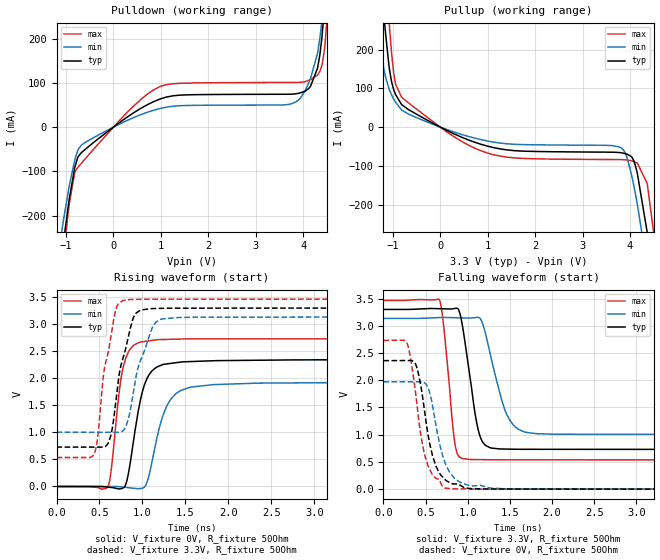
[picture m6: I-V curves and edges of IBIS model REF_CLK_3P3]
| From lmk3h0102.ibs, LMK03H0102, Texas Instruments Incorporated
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[Model]   REF_CLK_3P3
Model_type   Output
Polarity   Non-Inverting
Vmeas = 1.65
Vref = 0
Cref = 5pF
Rref = 100000
|   typ   min   max
C_comp   2.5pF   2pF   3pF
[Voltage Range]   3.3   3.135   3.465
[Temperature Range]   45   125   -40
[Pullup Reference]   3.3   3.135   3.465
[Pulldown Reference]   0   0   0
[Power Clamp Reference]   3.3   3.135   3.465
[GND Clamp Reference]   0   0   0
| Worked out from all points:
|   slope of the pulldown table from 0 to 0.495 V, typ, clamps not added: 13.4 ohm
|   slope of the pullup table from 0 to 0.495 V, typ, clamps not added: 17.5 ohm
|   falling waveform, V_fixture 3.3V, R_fixture 50Ohm: 20-80 % time 144ps typ, 214ps min, 103ps max; typ from 3.3 V to 0.729 V
|   rising waveform, V_fixture 0V, R_fixture 50Ohm: 20-80 % time 162ps typ, 202ps min, 119ps max; typ from 0 V to 2.35 V
|   rising waveform, V_fixture 3.3V, R_fixture 50Ohm: 20-80 % time 174ps typ, 203ps min, 151ps max; typ from 0.729 V to 3.3 V
|   falling waveform, V_fixture 0V, R_fixture 50Ohm: 20-80 % time 168ps typ, 180ps min, 161ps max; typ from 2.36 V to 0 V
[Pulldown]
|   Voltage   I(typ)   I(min)   I(max)
-3.3V     -2.545A    -2.251A    -2.867A
-1.063V   -267.1mA   -216mA     -295.7mA
-815.1mV  -90.95mA   -73.76mA   -101.8mA
-676.5mV  -57.76mA   -40.74mA   -81.81mA
986.7mV   63.7mA     42.19mA    91.87mA
3.759V    74.55mA    52.95mA    101mA
4.155V    92.27mA    109.9mA    107.6mA
4.303V    133.3mA    166.9mA    117.8mA
4.392V    200.1mA    237mA      138.6mA
4.452V    272.2mA    301.4mA    177.1mA
4.551V    422.3mA    428.4mA    315.2mA
6.6V      4.406A     3.787A     5.145A
[Pullup]
|   Voltage   I(typ)   I(min)   I(max)
-3.3V     4.359A     3.471A     5.492A
-1.33V    515.2mA    285mA      770.2mA
-1.171V   263.8mA    138mA      443.1mA
-1.073V   149.4mA    96.01mA    260.4mA
-943.8mV  84.25mA    64.34mA    111mA
-815.1mV  58.02mA    43.96mA    76.97mA
848.1mV   -43.87mA   -32.01mA   -60.5mA
3.798V    -65.86mA   -52.45mA   -83.74mA
4.085V    -88.71mA   -154.4mA   -89.1mA
4.363V    -271.7mA   -360.4mA   -145.4mA
4.689V    -576.5mA   -641.7mA   -450.2mA
6.6V      -2.525A    -2.382A    -2.651A
[Ramp]
R_load = 50
|   typ   min   max
dV/dt_r   1.40689/1.6153e-10   1.1607/2.0064e-10   1.63714/1.19152e-10
dV/dt_f   1.54251/1.44206e-10   1.27858/2.13592e-10   1.75671/1.02728e-10
[Falling Waveform]
V_fixture = 3.3V
V_fixture_min = 3.135V
V_fixture_max = 3.465V
R_fixture = 50Ohm
C_fixture = 0F
|   Time   V(typ)   V(min)   V(max)
0s        3.3V       3.135V     3.464V
666ps     3.313V     3.15V      3.469V
714.6ps   3.311V     3.153V     2.993V
842.3ps   3.317V     3.148V     898.2mV
926.3ps   3.093V     3.145V     568.3mV
1.12ns    1.115V     3.155V     543mV
1.26ns    763.5mV    2.527V     539.9mV
1.464ns   736mV      1.369V     538.9mV
1.685ns   732.1mV    1.047V     538.7mV
5ns       729mV      1.004V     536.4mV
[Rising Waveform]
V_fixture = 0V
V_fixture_min = 0V
V_fixture_max = 0V
R_fixture = 50Ohm
C_fixture = 0F
|   Time   V(typ)   V(min)   V(max)
0s        759.1nV    2.524uV    473.4nV
598.4ps   -11.6mV    -335uV     -6.053mV
638.3ps   -17.7mV    -357.5uV   330.6mV
769.4ps   -32.1mV    -10.13mV   2.159V
835.4ps   229.6mV    -21.49mV   2.481V
955.1ps   1.426V     -41.31mV   2.659V
1.077ns   2.065V     205.9mV    2.692V
1.289ns   2.267V     1.506V     2.719V
1.543ns   2.308V     1.828V     2.729V
5ns       2.345V     1.935V     2.729V
[Rising Waveform]
V_fixture = 3.3V
V_fixture_min = 3.135V
V_fixture_max = 3.465V
R_fixture = 50Ohm
C_fixture = 0F
|   Time   V(typ)   V(min)   V(max)
0s        728.9mV    1.004V     536.1mV
440.9ps   727.6mV    1.002V     614.4mV
481.6ps   727.5mV    1.002V     943.1mV
546.5ps   730.8mV    1.001V     2.06V
626.9ps   912.8mV    1.001V     2.713V
692.9ps   1.601V     1.001V     3.283V
769.4ps   2.349V     1.027V     3.434V
924.9ps   3.204V     2.023V     3.458V
1.217ns   3.292V     3.093V     3.462V
5ns       3.3V       3.134V     3.464V
[Falling Waveform]
|Gnd
V_fixture = 0V
V_fixture_min = 0V
V_fixture_max = 0V
R_fixture = 50Ohm
C_fixture = 0F
|   Time   V(typ)   V(min)   V(max)
0s        2.36V      1.97V      2.731V
282.3ps   2.362V     1.971V     2.674V
380ps     2.3V       1.971V     1.788V
442.5ps   1.906V     1.972V     1.004V
495.1ps   1.354V     1.941V     594.6mV
581.6ps   619.2mV    1.537V     266.8mV
724.4ps   188.4mV    514.6mV    24.95mV
911.3ps   71.44mV    124.3mV    5.016mV
1.269ns   2.743mV    20.49mV    2.336mV
5ns       181.4uV    170.4uV    158.4uV
